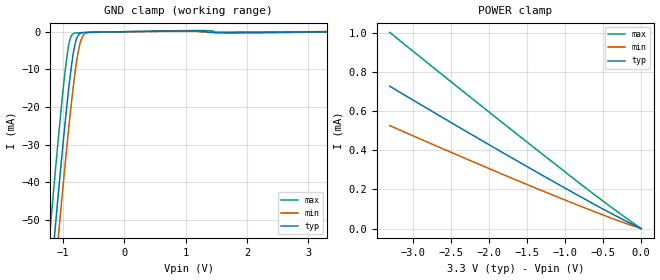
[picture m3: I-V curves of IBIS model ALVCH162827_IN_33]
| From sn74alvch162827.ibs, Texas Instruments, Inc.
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[Model]   ALVCH162827_IN_33
Model_type  Input
Vinl = 0.8
Vinh = 2.0
| variable   typ   min   max
C_comp   5.13pF   4.00pF   6.36pF
[Temperature Range]   40   100   -40
| Ambient temperature   25   85   -40
[Voltage range]   3.3   3   3.6
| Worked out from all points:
|   GND clamp passes 1 mA (typ) near -0.75 V on its own axis
[GND Clamp]
| ALVCH162827_IN_33
|   Voltage   I(typ)   I(min)   I(max)
-3.3V     -478.3mA   -488.4mA   -465.8mA
-1.215V   -69.66mA   -81.14mA   -54.95mA
-1.185V   -64.1mA    -75.59mA   -49.36mA
-1.125V   -53.1mA    -64.59mA   -38.36mA
-1.065V   -42.33mA   -53.77mA   -27.68mA
-925mV    -18.83mA   -29.68mA   -6.119mA
-875mV    -11.59mA   -21.75mA   -1.826mA
-820mV    -5.222mA   -13.81mA   -467uA
-770mV    -1.781mA   -7.751mA   -308.8uA
-715mV    -476.6uA   -3.105mA   -272.7uA
-585mV    -155.7uA   -203.6uA   -219.8uA
3.3V      8.676pA    40.66uA    -79.23uA
[POWER Clamp]
| ALVCH162827_IN_33
|   Voltage   I(typ)   I(min)   I(max)
-3.3V     726.6uA    525.7uA    1.001mA
-1.955V   418.9uA    299.6uA    582uA
-845mV    173.4uA    122.1uA    242.6uA
-430mV    85.18uA    59.36uA    120.2uA
-48.03fV  8.677pA    12.17pA    9.125pA
